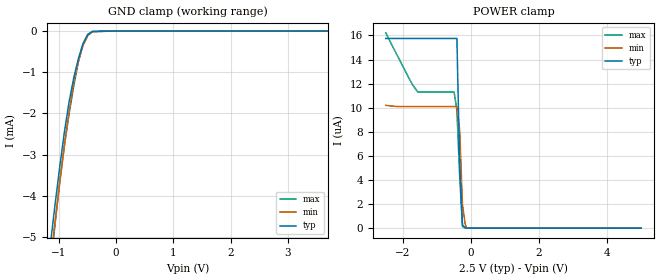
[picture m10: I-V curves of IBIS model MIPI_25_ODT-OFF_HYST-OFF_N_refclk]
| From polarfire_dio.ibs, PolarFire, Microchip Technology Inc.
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|   Model MIPI_25_ODT-OFF_HYST-OFF_N_refclk
[Model]   MIPI_25_ODT-OFF_HYST-OFF_N_refclk
Model_type   Input
Vinl =   1.125
Vinh =   1.375
|   typ   min   max
C_comp   2.671e-12   2.671e-12   2.761e-12
[Temperature Range]  25C   100C   -40C
[Voltage Range]  2.5   2.375   2.625
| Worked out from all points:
|   GND clamp passes 1 mA (typ) near -0.71 V on its own axis
[GND Clamp]
| Voltage   I(typ)   I(min)   I(max)
-2.5V     -29.41mA   -28.65mA   -32.17mA
-1.148V   -5.23mA    -5.664mA   -5.826mA
-1.066V   -4.254mA   -4.675mA   -4.737mA
-984.4mV  -3.331mA   -3.717mA   -3.705mA
-902.3mV  -2.478mA   -2.807mA   -2.8mA
-820.3mV  -1.738mA   -1.973mA   -2.031mA
-738.3mV  -1.148mA   -1.262mA   -1.341mA
-656.2mV  -667.7uA   -728.4uA   -750.3uA
-574.2mV  -304.1uA   -352.5uA   -314uA
-492.2mV  -84.33uA   -111.9uA   -81.65uA
-410.2mV  -8.903uA   -16.98uA   -8.141uA
5V        0A         0A         0A
[POWER Clamp]
| Voltage   I(typ)   I(min)   I(max)
-2.5V     15.76uA    10.21uA    16.22uA
-2.133V   15.76uA    10.1uA     14.18uA
-1.723V   15.76uA    10.1uA     11.95uA
-1.559V   15.76uA    10.1uA     11.31uA
-492.2mV  15.76uA    10.1uA     11.31uA
-410.2mV  15.76uA    10.1uA     9.823uA
-328.1mV  5.279uA    8.13uA     4.39uA
-246.1mV  272.1nA    1.95uA     119.3nA
-164.1mV  12.78nA    303.7nA    20.04nA
-125mV    9.473nA    47.11nA    20.04nA
-82.03mV  9.473nA    23.29nA    20.04nA
5V        0A         0A         0A
